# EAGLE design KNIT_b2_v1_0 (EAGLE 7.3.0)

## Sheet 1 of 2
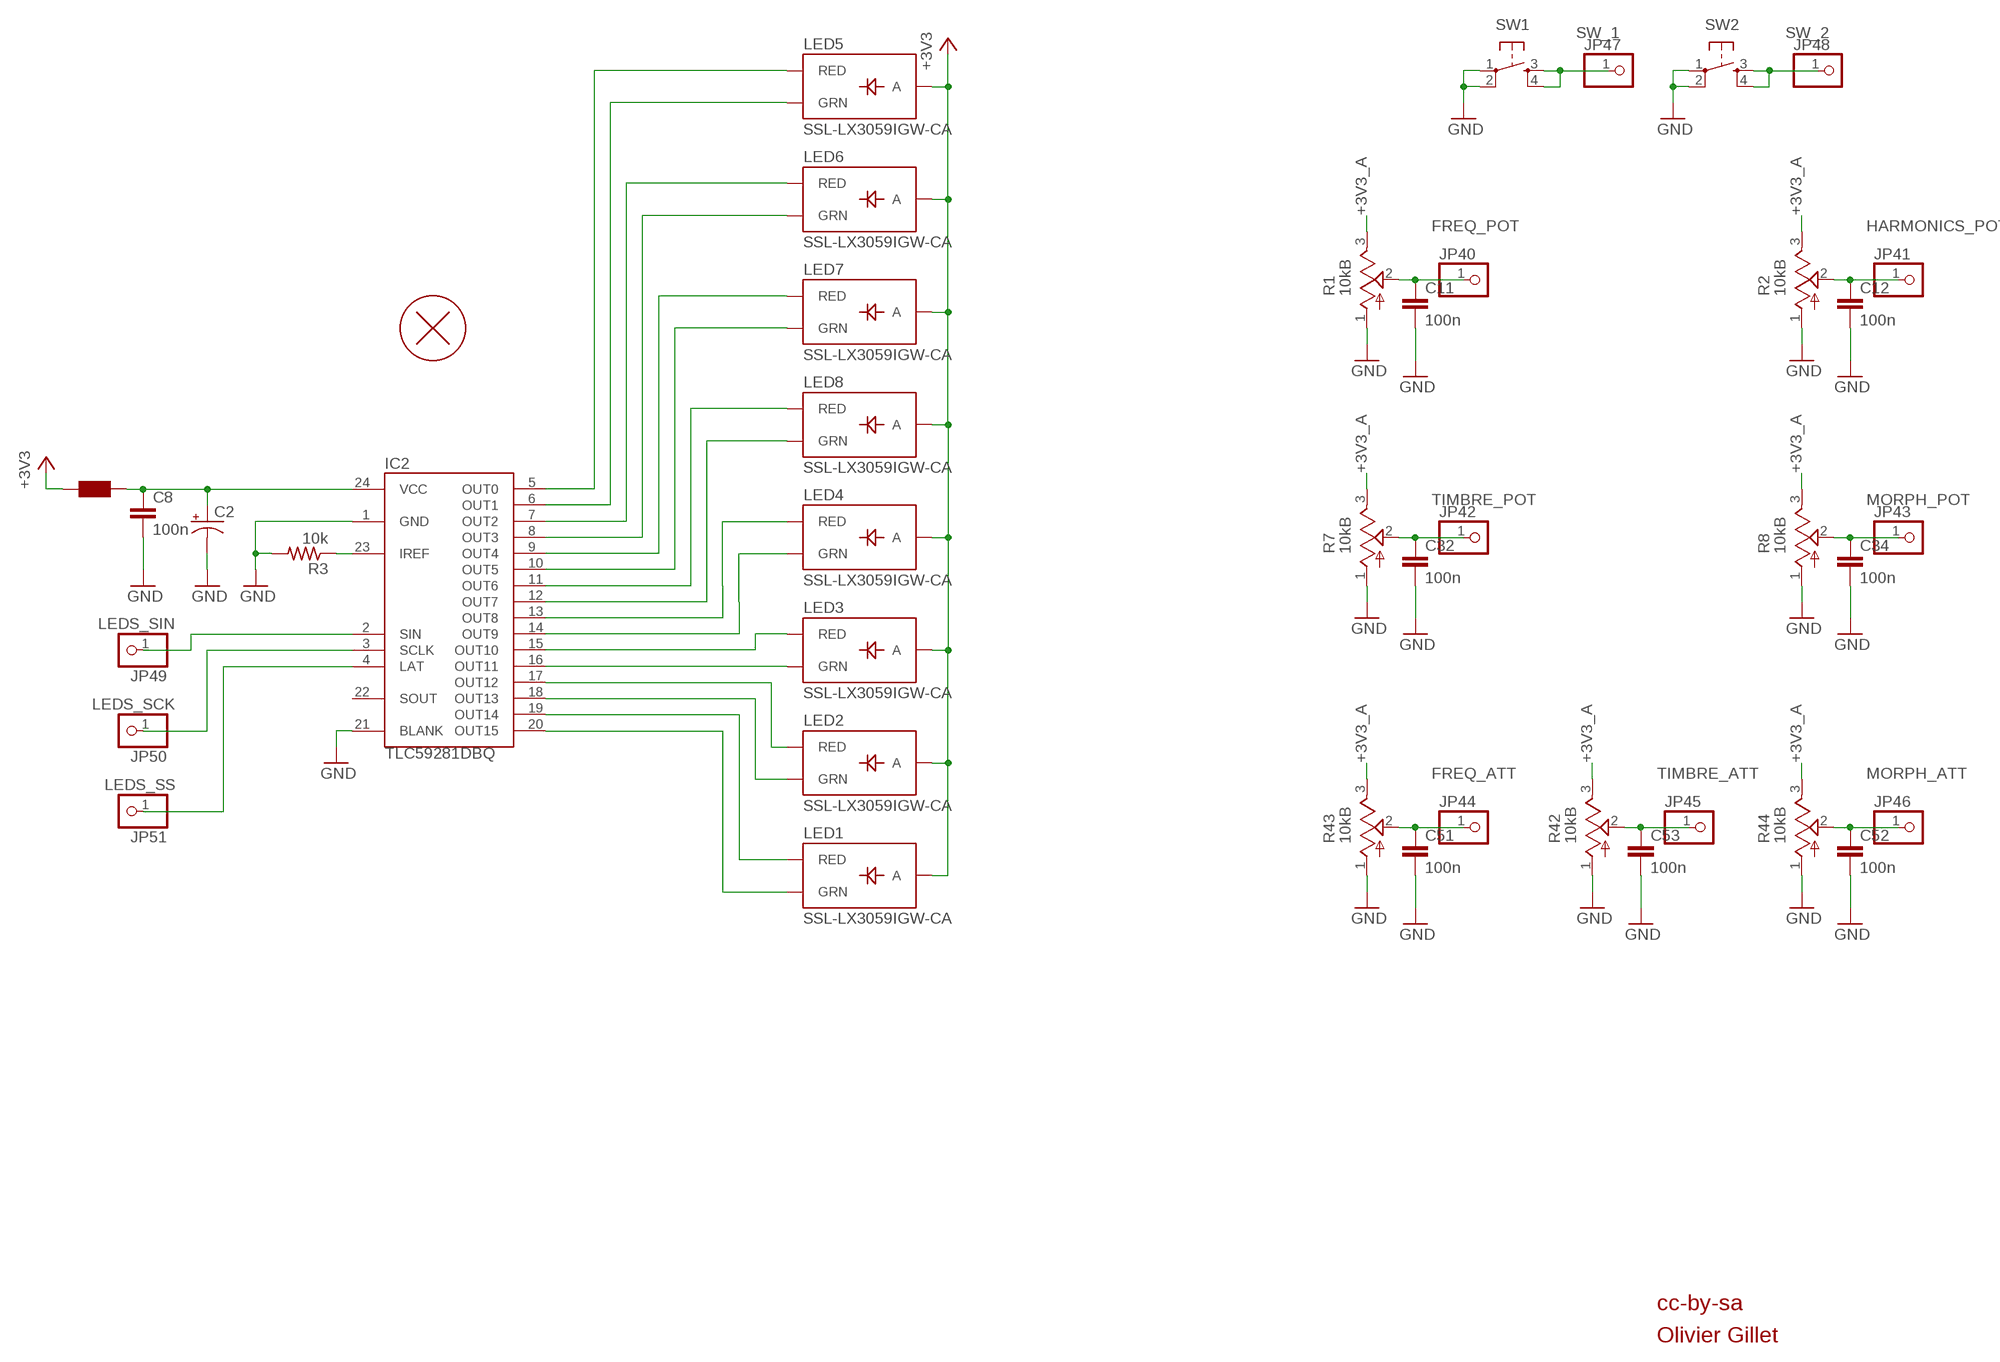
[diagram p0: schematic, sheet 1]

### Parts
C2  CAP_POL  [PANASONIC_B]
C8  100n  CAPACITOR  [RESISTOR_0603]
C11  100n  CAPACITOR  [RESISTOR_0603]
C12  100n  CAPACITOR  [RESISTOR_0603]
C32  100n  CAPACITOR  [RESISTOR_0603]
C34  100n  CAPACITOR  [RESISTOR_0603]
C51  100n  CAPACITOR  [RESISTOR_0603]
C52  100n  CAPACITOR  [RESISTOR_0603]
C53  100n  CAPACITOR  [RESISTOR_0603]
F1  FERRITE-BEAD  [RESISTOR_0603]
H1  PCB_SCREW  [PCB_SCREW]
IC2  TLC59281DBQ  [TSSOP24_0635]
JP40  PINHD-1X1  [1X01]
JP41  PINHD-1X1  [1X01]
JP42  PINHD-1X1  [1X01]
JP43  PINHD-1X1  [1X01]
JP44  PINHD-1X1  [1X01]
JP45  PINHD-1X1  [1X01]
JP46  PINHD-1X1  [1X01]
JP47  PINHD-1X1  [1X01]
JP48  PINHD-1X1  [1X01]
JP49  PINHD-1X1  [1X01]
JP50  PINHD-1X1  [1X01]
JP51  PINHD-1X1  [1X01]
LED1  SSL-LX3059IGW-CA  LED-BICOLOR-THROUGHHOLE-CA  [LED-BICOLOR-THROUGHHOLE-LUMEX]
LED2  SSL-LX3059IGW-CA  LED-BICOLOR-THROUGHHOLE-CA  [LED-BICOLOR-THROUGHHOLE-LUMEX]
LED3  SSL-LX3059IGW-CA  LED-BICOLOR-THROUGHHOLE-CA  [LED-BICOLOR-THROUGHHOLE-LUMEX]
LED4  SSL-LX3059IGW-CA  LED-BICOLOR-THROUGHHOLE-CA  [LED-BICOLOR-THROUGHHOLE-LUMEX]
LED5  SSL-LX3059IGW-CA  LED-BICOLOR-THROUGHHOLE-CA  [LED-BICOLOR-THROUGHHOLE-LUMEX]
LED6  SSL-LX3059IGW-CA  LED-BICOLOR-THROUGHHOLE-CA  [LED-BICOLOR-THROUGHHOLE-LUMEX]
LED7  SSL-LX3059IGW-CA  LED-BICOLOR-THROUGHHOLE-CA  [LED-BICOLOR-THROUGHHOLE-LUMEX]
LED8  SSL-LX3059IGW-CA  LED-BICOLOR-THROUGHHOLE-CA  [LED-BICOLOR-THROUGHHOLE-LUMEX]
R1  10kB  POT_VERTICAL  [ALPS_POT_VERTICAL]
R2  10kB  POT_VERTICAL  [ALPS_POT_VERTICAL]
R3  10k  RESISTOR  [RESISTOR_0603]
R7  10kB  POT_VERTICAL  [ALPS_POT_VERTICAL]
R8  10kB  POT_VERTICAL  [ALPS_POT_VERTICAL]
R42  10kB  POT_VERTICAL  [ALPS_POT_VERTICAL]
R43  10kB  POT_VERTICAL  [ALPS_POT_VERTICAL]
R44  10kB  POT_VERTICAL  [ALPS_POT_VERTICAL]
SW1  TAC_SWITCHPTH  [TACTILE-PTH]
SW2  TAC_SWITCHPTH  [TACTILE-PTH]

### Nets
+3V3: F1.2 LED1.A LED2.A LED3.A LED4.A LED5.A LED6.A LED7.A LED8.A ; also sheet 2
+3V3_A: R1.3(B) R2.3(B) R7.3(B) R8.3(B) R42.3(B) R43.3(B) R44.3(B) ; also sheet 2
FREQ_ATT: C51.1 JP44.1 R43.2(W)
FREQ_POT: C11.1 JP40.1 R1.2(W)
GND: C2.- C8.2 C11.2 C12.2 C32.2 C34.2 C51.2 C52.2 C53.2 IC2.1(GND) IC2.21(BLANK) R1.1(A) R2.1(A) R3.2 R7.1(A) R8.1(A) R42.1(A) R43.1(A) R44.1(A) SW1.1 SW1.2 SW2.1 SW2.2 ; also sheet 2
HARMONICS_POT: C12.1 JP41.1 R2.2(W)
LEDS_SCK: IC2.3(SCLK) JP50.1
LEDS_SIN: IC2.2(SIN) JP49.1
LEDS_SS: IC2.4(LAT) JP51.1
MORPH_ATT: C52.1 JP46.1 R44.2(W)
MORPH_POT: C34.1 JP43.1 R8.2(W)
N$2: IC2.12(OUT7) LED8.GREEN_C(GRN)
N$5: IC2.11(OUT6) LED8.RED_C(RED)
N$9: IC2.10(OUT5) LED7.GREEN_C(GRN)
N$10: IC2.9(OUT4) LED7.RED_C(RED)
N$11: IC2.8(OUT3) LED6.GREEN_C(GRN)
N$12: IC2.13(OUT8) LED4.RED_C(RED)
N$13: IC2.7(OUT2) LED6.RED_C(RED)
N$14: IC2.14(OUT9) LED4.GREEN_C(GRN)
N$15: IC2.6(OUT1) LED5.GREEN_C(GRN)
N$17: IC2.15(OUT10) LED3.RED_C(RED)
N$18: IC2.16(OUT11) LED3.GREEN_C(GRN)
N$19: IC2.17(OUT12) LED2.RED_C(RED)
N$20: IC2.18(OUT13) LED2.GREEN_C(GRN)
N$21: IC2.19(OUT14) LED1.RED_C(RED)
N$22: IC2.5(OUT0) LED5.RED_C(RED)
N$23: IC2.20(OUT15) LED1.GREEN_C(GRN)
N$27: C2.+ C8.1 F1.1 IC2.24(VCC)
N$68: IC2.23(IREF) R3.1
SW_1: JP47.1 SW1.3 SW1.4
SW_2: JP48.1 SW2.3 SW2.4
TIMBRE_ATT: C53.1 JP45.1 R42.2(W)
TIMBRE_POT: C32.1 JP42.1 R7.2(W)
Unconnected: IC2.22(SOUT)

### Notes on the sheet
- cc-by-sa
- Olivier Gillet

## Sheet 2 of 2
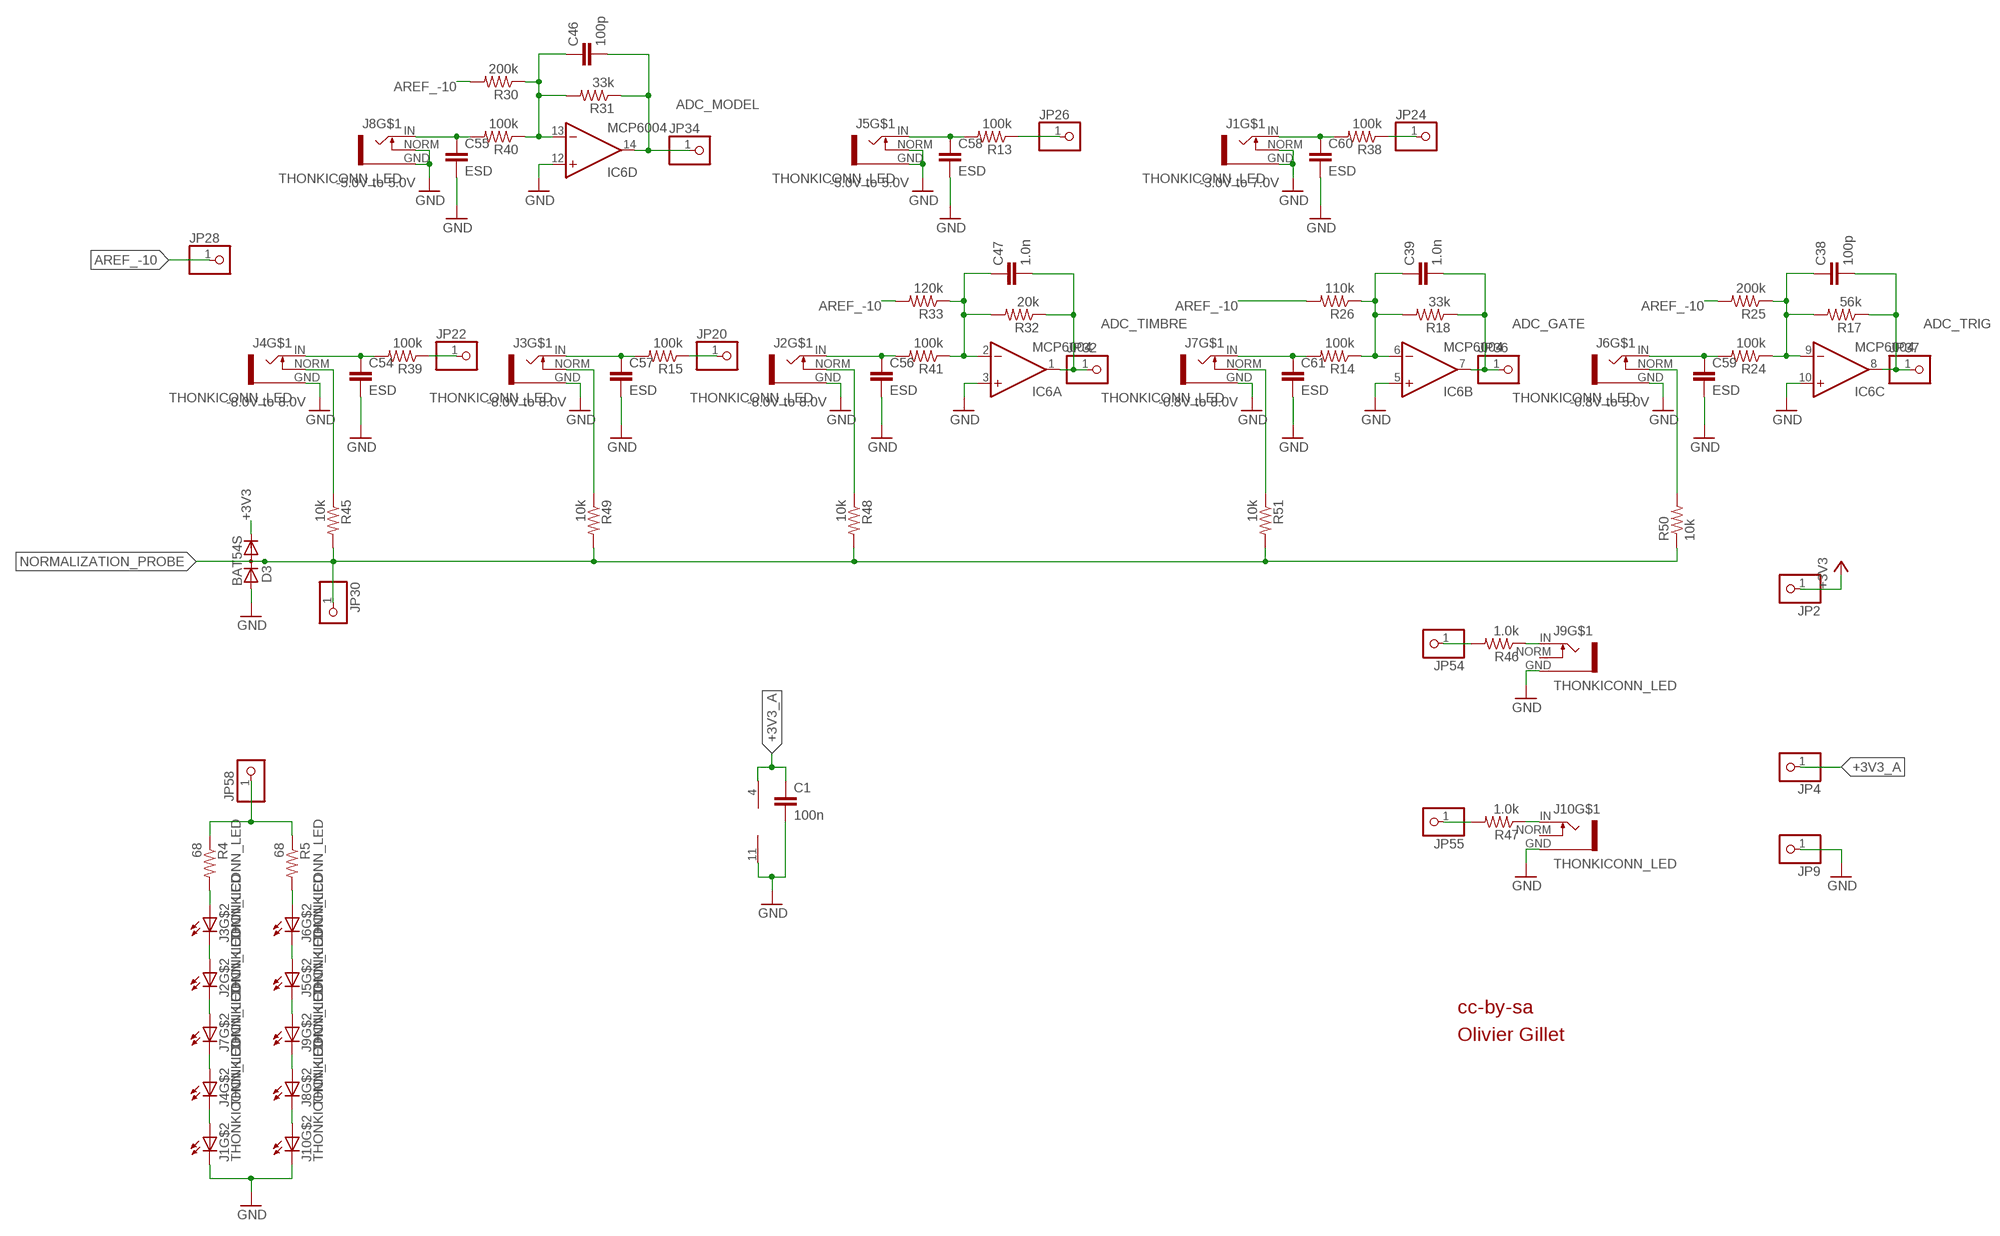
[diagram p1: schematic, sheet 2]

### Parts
C1  100n  CAPACITOR  [RESISTOR_0603]
C38  100p  CAPACITOR  [RESISTOR_0603]
C39  1.0n  CAPACITOR  [RESISTOR_0603]
C46  100p  CAPACITOR  [RESISTOR_0603]
C47  1.0n  CAPACITOR  [RESISTOR_0603]
C54  ESD  CAPACITOR  [RESISTOR_0603]
C55  ESD  CAPACITOR  [RESISTOR_0603]
C56  ESD  CAPACITOR  [RESISTOR_0603]
C57  ESD  CAPACITOR  [RESISTOR_0603]
C58  ESD  CAPACITOR  [RESISTOR_0603]
C59  ESD  CAPACITOR  [RESISTOR_0603]
C60  ESD  CAPACITOR  [RESISTOR_0603]
C61  ESD  CAPACITOR  [RESISTOR_0603]
D3  BAT54S  DIODE_2CACA-SOT23  [SOT23]
IC6  MCP6004  TL074PW  [TSSOP14_065]
J1  THONKICONN_LED  [LED_JACK]
J2  THONKICONN_LED  [LED_JACK]
J3  THONKICONN_LED  [LED_JACK]
J4  THONKICONN_LED  [LED_JACK]
J5  THONKICONN_LED  [LED_JACK]
J6  THONKICONN_LED  [LED_JACK]
J7  THONKICONN_LED  [LED_JACK]
J8  THONKICONN_LED  [LED_JACK]
J9  THONKICONN_LED  [LED_JACK]
J10  THONKICONN_LED  [LED_JACK]
JP2  PINHD-1X1  [1X01]
JP4  PINHD-1X1  [1X01]
JP9  PINHD-1X1  [1X01]
JP20  PINHD-1X1  [1X01]
JP22  PINHD-1X1  [1X01]
JP24  PINHD-1X1  [1X01]
JP26  PINHD-1X1  [1X01]
JP28  PINHD-1X1  [1X01]
JP30  PINHD-1X1  [1X01]
JP32  PINHD-1X1  [1X01]
JP34  PINHD-1X1  [1X01]
JP36  PINHD-1X1  [1X01]
JP37  PINHD-1X1  [1X01]
JP54  PINHD-1X1  [1X01]
JP55  PINHD-1X1  [1X01]
JP58  PINHD-1X1  [1X01]
R4  68  RESISTOR  [RESISTOR_0603]
R5  68  RESISTOR  [RESISTOR_0603]
R13  100k  RESISTOR  [RESISTOR_0603]
R14  100k  RESISTOR  [RESISTOR_0603]
R15  100k  RESISTOR  [RESISTOR_0603]
R17  56k  RESISTOR  [RESISTOR_0603]
R18  33k  RESISTOR  [RESISTOR_0603]
R24  100k  RESISTOR  [RESISTOR_0603]
R25  200k  RESISTOR  [RESISTOR_0603]
R26  110k  RESISTOR  [RESISTOR_0603]
R30  200k  RESISTOR  [RESISTOR_0603]
R31  33k  RESISTOR  [RESISTOR_0603]
R32  20k  RESISTOR  [RESISTOR_0603]
R33  120k  RESISTOR  [RESISTOR_0603]
R38  100k  RESISTOR  [RESISTOR_0603]
R39  100k  RESISTOR  [RESISTOR_0603]
R40  100k  RESISTOR  [RESISTOR_0603]
R41  100k  RESISTOR  [RESISTOR_0603]
R45  10k  RESISTOR  [RESISTOR_0603]
R46  1.0k  RESISTOR  [RESISTOR_0603]
R47  1.0k  RESISTOR  [RESISTOR_0603]
R48  10k  RESISTOR  [RESISTOR_0603]
R49  10k  RESISTOR  [RESISTOR_0603]
R50  10k  RESISTOR  [RESISTOR_0603]
R51  10k  RESISTOR  [RESISTOR_0603]

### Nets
+3V3: D3.2(C) JP2.1 ; also sheet 1
+3V3_A: C1.1 IC6.4(P:V+) JP4.1 ; also sheet 1
ADC_GATE: C39.2 IC6.7(B:OUT) JP36.1 R18.1
ADC_MODEL: C46.2 IC6.14(D:OUT) JP34.1 R31.1
ADC_TIMBRE: C47.2 IC6.1(A:OUT) JP32.1 R32.1
ADC_TRIG: C38.2 IC6.8(C:OUT) JP37.1 R17.1
AREF_-10: JP28.1 R25.2 R26.2 R30.2 R33.2
FM_IN: C57.1 J3.IN R15.2
GATE_IN: C61.1 J7.IN R14.2
GATE_IN1: C59.1 J6.IN R24.2
GND: C1.2 C54.2 C55.2 C56.2 C57.2 C58.2 C59.2 C60.2 C61.2 D3.1(A) IC6.3(A:+IN) IC6.5(B:+IN) IC6.10(C:+IN) IC6.11(P:V-) IC6.12(D:+IN) J1.C J1.GND J1.NORM J2.GND J3.GND J4.GND J5.GND J5.NORM J6.GND J7.GND J8.GND J8.NORM J9.GND J10.C J10.GND JP9.1 ; also sheet 1
HARMONICS_IN: C58.1 J5.IN R13.2
MODEL_IN: C55.1 J8.IN R40.2
MORPH_IN: C54.1 J4.IN R39.2
N$1: J2.A J3.C
N$3: J6.NORM R50.2
N$4: C38.1 IC6.9(C:-IN) R17.2 R24.1 R25.1
N$6: J2.C J7.A
N$7: J4.A J7.C
N$8: J1.A J4.C
N$16: J5.A J6.C
N$24: J3.NORM R49.1
N$25: J2.NORM R48.1
N$26: J4.NORM R45.1
N$28: C39.1 IC6.6(B:-IN) R14.1 R18.2 R26.1
N$29: J5.C J9.A
N$30: J8.A J9.C
N$31: C56.1 J2.IN R41.2
N$32: J8.C J10.A
N$33: J3.A R4.2
N$34: J6.A R5.2
N$35: JP58.1 R4.1 R5.1
N$36: J7.NORM R51.1
N$37: C46.1 IC6.13(D:-IN) R30.1 R31.2 R40.1
N$39: C47.1 IC6.2(A:-IN) R32.2 R33.1 R41.1
N$44: JP20.1 R15.1
N$45: JP22.1 R39.1
N$49: JP24.1 R38.1
N$50: JP26.1 R13.1
N$52: JP54.1 R46.2
N$53: JP55.1 R47.2
N$65: J9.IN R46.1
N$69: J10.IN R47.1
NORMALIZATION_PROBE: D3.3(AC) JP30.1 R45.2 R48.2 R49.2 R50.1 R51.2
V_OCT_IN: C60.1 J1.IN R38.2
Unconnected: J9.NORM J10.NORM

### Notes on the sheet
- -5.0V to 5.0V | -5.0V to 5.0V | -3.0V to 7.0V
- -8.0V to 8.0V | -8.0V to 8.0V | -8.0V to 8.0V | -0.8V to 8.0V | -0.8V to 5.0V
- cc-by-sa
- Olivier Gillet

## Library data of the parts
C1 C8 C11 C12 C32 C34 C38 C39 C46 C47 C51-C61 = parts_aman:CAPACITOR
C2 = parts_aman:CAP_POL
D3 = diode:DIODE_2CACA-: 2 Diodes - Cathode-Anode|Cathode-Anode
F1 = parts_aman:FERRITE-BEAD
H1 = parts_aman:PCB_SCREW
IC2 = og-ics:TLC59281
IC6 = og-linear:TL074: OP AMP
J1-J10 = parts_aman:THONKICONN_LED
JP2 JP4 JP9 JP20 JP22 JP24 JP26 JP28 JP30 JP32 JP34 JP36 JP37 JP40-JP51 JP54 JP55 JP58 = parts_aman:PINHD-1X1: PIN HEADER
LED1-LED8 = og-leds:LED-BICOLOR-THROUGHHOLE-CA
R1 R2 R7 R8 R42-R44 = parts_aman:POT_VERTICAL
R3-R5 R13-R15 R17 R18 R24-R26 R30-R33 R38-R41 R45-R51 = parts_aman:RESISTOR
SW1 SW2 = SparkFun:TAC_SWITCH: Momentary Switch Button commonly used for reset or general input. Spark Fun Electronics SKU : COM-00097

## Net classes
0 default: width 0.152 mm, drill 0.305 mm, clearance 0.152 mm

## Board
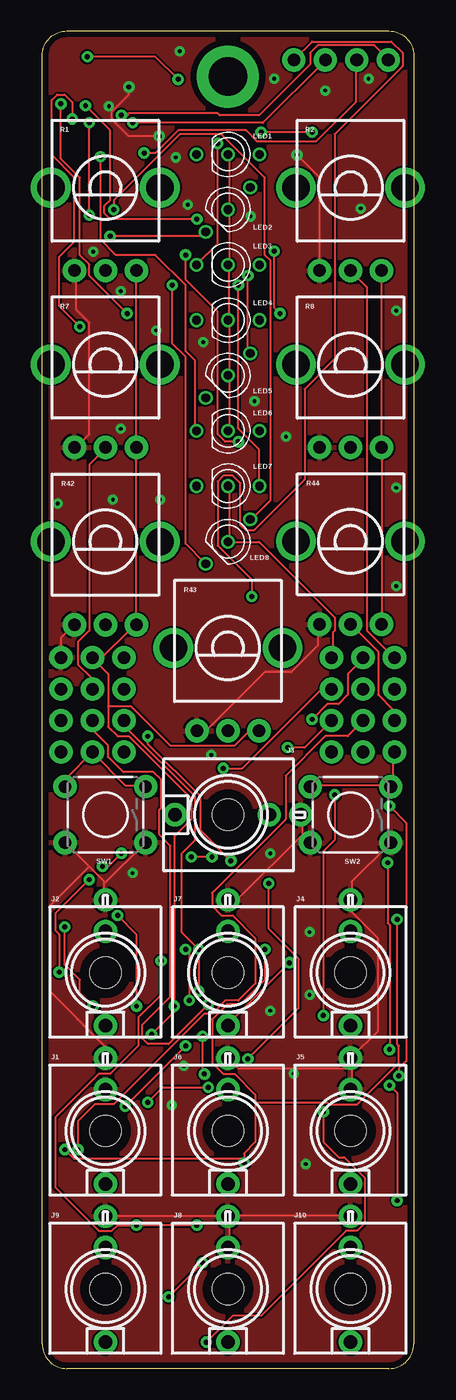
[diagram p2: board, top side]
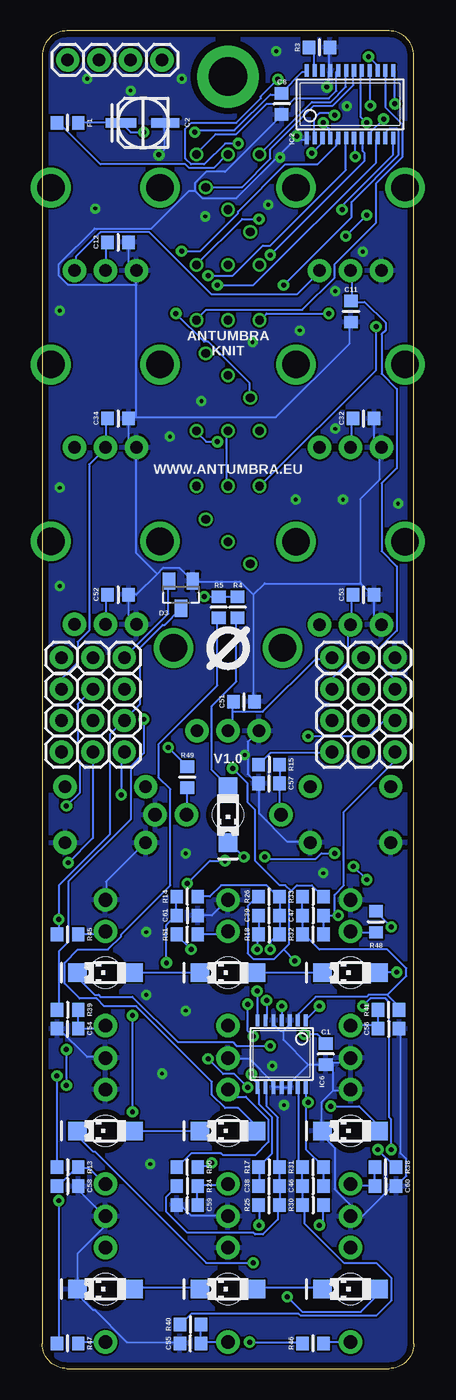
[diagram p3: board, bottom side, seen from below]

Size 30 x 108 mm. Coordinates in mm from the lower left corner, seen from the top.
Outline: 28,0 2,0 arc-90 0,2 0,106 arc-90 2,108 28,108 arc-90 30,106 30,2 arc-90 28,0
Copper layers (1*16): Top 0.035mm / dielectric 1.5mm / Bottom 0.035mm
Design rules "PCBCart-Standard *": minimum track width 6mil, minimum drill 0.4mm, track to track 6mil, track to pad 6mil, pad to pad 6mil, via to via 6mil, smd to smd 6mil, copper to edge 20mil, drill to drill 8mil, minimum pad ring 8mil, minimum via ring 10mil, stop-mask expansion 3mil, vias tented up to drill 25mil, thermal gap 8mil

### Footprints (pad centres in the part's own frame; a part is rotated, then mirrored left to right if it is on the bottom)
RESISTOR_0603 = smd 1 x 1.1: 1 -0.85,0; 2 0.85,0
PANASONIC_B = smd 2.464 x 0.762: + 1.778,0 | smd 2.286 x 0.762: - -1.778,0
SOT23 = smd 1 x 1.4: 1 -0.95,-1.1; 2 0.95,-1.1; 3 0,1.1
PCB_SCREW = drill 3.1 pad 5: P$1 0,0
TSSOP24_0635 = smd 0.33 x 1: 1 -3.493,-2.725; 2 -2.857,-2.725; 3 -2.223,-2.725; 4 -1.587,-2.725; 5 -0.953,-2.725; 6 -0.318,-2.725; 7 0.318,-2.725; 8 0.953,-2.725; 9 1.587,-2.725; 10 2.223,-2.725; 11 2.857,-2.725; 12 3.493,-2.725; 13 3.493,2.725; 14 2.857,2.725; 15 2.223,2.725; 16 1.587,2.725; 17 0.953,2.725; 18 0.318,2.725; 19 -0.318,2.725; 20 -0.953,2.725; 21 -1.587,2.725; 22 -2.223,2.725; 23 -2.857,2.725; 24 -3.493,2.725
TSSOP14_065 = smd 0.305 x 0.991: 1 -1.95,-2.718; 2 -1.3,-2.718; 3 -0.65,-2.718; 4 0,-2.718; 5 0.65,-2.718; 6 1.3,-2.718; 7 1.95,-2.718; 8 1.95,2.718; 9 1.3,2.718; 10 0.65,2.718; 11 0,2.718; 12 -0.65,2.718; 13 -1.3,2.718; 14 -1.95,2.718
LED_JACK = smd 1.5 x 1.5 bottom: A 2.266,0; C -2.266,0 | drill 1.1 pad 1.88: GND 0,-5.88; IN 0,4.28; NORM 0,-3.34 | hole 2.5: 0,0
1X01 = drill 1.016 pad 1.88: 1 0,0
LED-BICOLOR-THROUGHHOLE-LUMEX = drill 0.7: A 0,0; GREEN_C 2.54,0; RED_C -2.54,0
ALPS_POT_VERTICAL = drill 1 pad 1.88: 1 -2.5,-6.7; 2 0,-6.7; 3 2.5,-6.7 | drill 2.2 pad 3.175: P$4 4.4,0; P$5 -4.4,0
TACTILE-PTH = drill 1.016 pad 1.88: 1 -3.251,2.261; 2 3.251,2.261; 3 -3.251,-2.261; 4 3.251,-2.261

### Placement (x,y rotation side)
C1  7.11,25.4 270 bottom
C2  21.84,100.58 180 bottom
C8  10.67,102.11 270 bottom
C11  5.08,85.34 270 bottom
C12  23.88,90.93 0 bottom
C32  4.06,76.71 0 bottom
C34  23.88,76.71 0 bottom
C38  11.68,14.73 180 bottom
C39  11.68,36.58 180 bottom
C46  8.13,14.73 0 bottom
C47  8.13,36.58 0 bottom
C51  13.72,53.85 0 bottom
C52  23.88,62.48 0 bottom
C53  4.06,62.48 0 bottom
C54  27.94,27.43 180 bottom
C55  18.03,2.03 180 bottom
C56  2.03,27.43 0 bottom
C57  11.68,47.24 180 bottom
C58  27.94,14.73 0 bottom
C59  18.29,13.21 180 bottom
C60  2.29,14.73 0 bottom
C61  18.29,36.58 0 bottom
D3  18.8,62.48 180 bottom
F1  27.94,100.58 180 bottom
H1  15,104.31 0 top
IC2  5.15,102.08 0 bottom
IC6  10.67,25.4 180 bottom
J1  5.11,19.19 180 top
J2  5.11,31.96 180 top
J3  15,44.71 90 top
J4  24.89,31.96 180 top
J5  24.89,19.19 180 top
J6  15,19.19 180 top
J7  15,31.96 180 top
J8  15,6.42 180 top
J9  5.11,6.42 180 top
J10  24.89,6.42 180 top
JP2  23.37,57.4 0 bottom
JP4  4.06,57.4 0 bottom
JP9  1.52,57.4 0 bottom
JP20  6.6,49.78 0 bottom
JP22  25.91,57.4 0 bottom
JP24  25.91,52.32 0 bottom
JP26  25.91,54.86 0 bottom
JP28  23.37,54.86 0 bottom
JP30  23.37,52.32 0 bottom
JP32  1.52,49.78 0 bottom
JP34  1.52,52.32 0 bottom
JP36  6.6,52.32 0 bottom
JP37  4.06,52.32 0 bottom
JP40  1.52,54.86 0 bottom
JP41  28.45,57.4 0 bottom
JP42  4.06,54.86 0 bottom
JP43  28.45,54.86 0 bottom
JP44  6.6,57.4 0 bottom
JP45  6.6,54.86 0 bottom
JP46  28.45,52.32 0 bottom
JP47  4.06,49.78 0 bottom
JP48  28.45,49.78 0 bottom
JP49  27.94,105.66 0 bottom
JP50  25.4,105.66 0 bottom
JP51  22.86,105.66 0 bottom
JP54  23.37,49.78 0 bottom
JP55  25.91,49.78 0 bottom
JP58  20.32,105.66 0 bottom
LED1  15,98.04 0 top
LED2  15,93.58 45 top
LED3  15,89.11 0 top
LED4  15,84.65 0 top
LED5  15,80.18 45 top
LED6  15,75.72 0 top
LED7  15,71.26 0 top
LED8  15,66.76 45 top
R1  5.11,95.35 0 top
R2  24.89,95.35 0 top
R3  7.62,106.68 0 bottom
R4  14.22,61.47 270 bottom
R5  15.75,61.47 270 bottom
R7  5.11,81.07 0 top
R8  24.89,81.07 0 top
R13  27.94,16.26 0 bottom
R14  18.29,38.1 180 bottom
R15  11.68,48.77 0 bottom
R17  11.68,16.26 0 bottom
R18  11.68,35.05 0 bottom
R24  18.29,14.73 0 bottom
R25  11.68,13.21 180 bottom
R26  11.68,38.1 180 bottom
R30  8.13,13.21 0 bottom
R31  8.13,16.26 180 bottom
R32  8.13,35.05 180 bottom
R33  8.13,38.1 0 bottom
R38  2.29,16.26 180 bottom
R39  27.94,28.96 0 bottom
R40  18.03,3.56 0 bottom
R41  2.03,28.96 180 bottom
R42  5.11,66.76 0 top
R43  15,58.19 0 top
R44  24.89,66.79 0 top
R45  27.94,35.05 180 bottom
R46  8.13,2.03 180 bottom
R47  27.94,2.03 180 bottom
R48  3.05,36.07 90 bottom
R49  18.29,47.75 90 bottom
R50  18.29,16.26 180 bottom
R51  18.29,35.05 180 bottom
SW1  5.11,44.73 180 top
SW2  24.89,44.71 180 top
U$1  [LOGO_3.5]  14.99,58.17 0 bottom

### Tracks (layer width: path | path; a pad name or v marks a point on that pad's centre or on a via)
+3V3
  Top 0.152: LED7.A 15.09,71.17 15.09,66.9 LED8.A 15.09,66.75 17.53,66.75 23.62,60.66 23.62,59.59 23.47,59.44 23.47,57.45 JP2.1 | LED1.A 15.09,97.99 15.09,93.73 LED2.A 15.09,93.57 15.09,89.15 LED3.A 15.09,89 15.09,84.73 LED4.A 15.09,84.58 15.09,80.31 LED5.A 15.09,80.16 15.09,75.74 LED6.A
  Bottom 0.152: JP2.1 19.81,60.96 19.81,63.55 D3.2 | LED6.A 15.09,75.59 15.09,71.32 LED7.A | F1.2 28.65,100.58 25.3,97.23 18.44,97.23 18.14,96.93 16.15,96.93 15.09,97.99 LED1.A
+3V3_A  (via drill 0.4)
  Top 0.152: R44.3 27.43,60.2 27.43,74.22 R8.3 27.43,74.37 27.43,88.54 R2.3 | v8.84,26.98 10.67,28.8 v10.67,29.26 10.67,42.98 12.04,44.35 12.04,46.02 7.01,51.05 6.1,51.05 5.33,51.82 5.33,53.49 | 5.33,53.49 5.33,56.08 4.42,57 | 4.42,57 4.12,57.3 JP4.1 4.42,57 | 4.42,57 7.47,60.05 R42.3 7.62,60.2 7.62,74.22 R7.3 7.62,88.54 R1.3 | 5.33,53.49 7.16,53.49 10.36,50.29 15.54,50.29 16.61,51.36 17.37,51.36 R43.3
  Bottom 0.152: v10.67,29.26 IC6.4 | v8.84,26.98 7.77,26.98 7.16,26.36 C1.1 | R2.3 27.28,88.7 27.28,89.76 25.3,91.75 21.34,91.75 16.31,86.72 9.45,86.72 7.62,88.54 R1.3
ADC_GATE  (via drill 0.4)
  Top 0.152: v12.65,30.48 v12.65,33.83 11.28,35.2 11.28,41.6 12.34,42.67 12.34,46.18 6.71,51.82 6.71,52.27 JP36.1
  Bottom 0.152: v12.65,30.48 12.65,28.19 IC6.7 | v12.65,33.83 12.65,35.05 R18.1 12.5,35.05 12.5,36.58 C39.2
ADC_MODEL  (via drill 0.4)
  Top 0.152: v8.53,51.05 8.53,50.44 12.8,46.18 12.8,43.43 v15.24,41 | v18.29,39.17 18.29,35.51 20.73,33.07 20.73,29.11 v16.61,24.99 | v13.41,22.71 9.75,22.71 v8.53,21.49
  Bottom 0.152: 8.69,21.49 8.69,17.68 7.32,16.31 R31.1 7.32,16.15 7.32,14.78 C46.2 | 8.69,21.49 8.69,22.55 IC6.14 | v8.53,51.05 3.66,51.05 2.44,52.27 1.52,52.27 JP34.1 | v15.24,41 16.46,41 v18.29,39.17 | v16.61,24.99 15.39,23.77 14.48,23.77 v13.41,22.71 | 8.69,21.49 v8.53,21.49
ADC_TIMBRE  (via drill 0.4)
  Top 0.152: v7.62,29.26 7.62,35.05 v6.1,36.58
  Bottom 0.152: v7.62,29.26 8.69,28.19 IC6.1 | 6.4,36.58 C47.2 7.32,36.58 7.32,35.05 R32.1 | JP32.1 1.52,49.07 5.64,44.96 5.64,39.01 6.4,38.25 6.4,36.58 | 6.4,36.58 v6.1,36.58
ADC_TRIG  (via drill 0.4)
  Top 0.152: v13.41,29.41 10.21,26.21 8.53,26.21 8.08,26.67 8.08,27.74 10.36,30.02 10.36,42.22 9.45,43.13 9.45,45.11 9.6,45.26 9.6,47.55 8.99,48.16 6.55,48.16 5.33,49.38 5.33,50.29 4.12,51.51 4.12,52.27 JP37.1 | v12.95,26.82 12.95,23.93 v13.11,23.77
  Bottom 0.152: C38.2 12.5,14.78 12.5,16.15 R17.1 12.5,16.31 11.43,17.37 11.43,20.27 12.5,21.34 12.5,22.55 IC6.8 12.65,22.71 12.65,23.01 13.11,23.47 v13.11,23.77 | v13.41,29.41 13.41,27.28 v12.95,26.82
AREF_-10  (via drill 0.4)
  Top 0.152: v12.5,11.58 v7.62,11.58 6.1,11.58 5.64,11.12 4.57,11.12 1.07,14.63 1.07,20.27 4.57,23.77 5.49,23.77 7.77,26.06 7.77,28.35 9.6,30.18 v9.6,32.92 | JP28.1 22.55,54.86 16.15,48.46 v14.63,48.46
  Bottom 0.152: v7.62,11.58 7.32,11.89 7.32,13.11 R30.2 | v12.5,11.58 12.5,13.11 R25.2 | 9.91,38.56 10.06,38.41 10.06,34.29 10.52,33.83 | 9.91,38.56 9.45,39.01 8.23,39.01 7.32,38.1 R33.2 | 10.52,33.83 11.28,33.07 12.95,33.07 13.41,33.53 13.41,37.34 12.65,38.1 R26.2 | 10.52,33.83 v9.6,32.92 | v14.63,48.46 13.41,47.24 13.41,45.72 12.8,45.11 12.8,41 10.82,39.01 10.36,39.01 9.91,38.56
FM_IN
  Bottom 0.152: C57.1 R15.2 | C57.1 10.82,44.81 J3.IN | C57.1
FREQ_ATT
  Bottom 0.152: 14.63,53.03 14.63,51.82 14.94,51.51 R43.2 | 14.63,53.03 14.63,53.8 C51.1 | 14.63,53.03 12.19,53.03 7.92,57.3 6.71,57.3 JP44.1
FREQ_POT
  Bottom 0.152: R1.2 5.03,88.54 5.03,86.26 C11.1 5.03,86.11 3.96,86.11 2.29,84.43 2.29,83.82 2.59,83.52 2.59,80.31 1.37,79.1 1.37,72.69 2.59,71.48 2.59,65.99 1.37,64.77 1.37,59.59 2.74,58.22 2.74,56.84 1.52,55.63 JP40.1
GATE_IN  (via drill 0.4)
  Top 0.152: v19.96,32.77 14.94,27.74 J7.IN
  Bottom 0.152: 19.2,36.58 19.2,38.1 R14.2 | 19.2,36.58 19.96,35.81 v19.96,32.77 | 19.2,36.58 C61.1
GATE_IN1
  Bottom 0.152: C59.1 17.53,13.26 17.53,14.63 R24.2 17.37,14.78 15.09,14.78 J6.IN
GND  (via drill 0.3, 0.4)
  Top 0.152: SW2.1 28.04,42.37 24.99,39.32 24.99,37.95 J4.GND 24.99,37.8 24.99,36.88 27.13,34.75 27.13,27.28 24.99,25.15 J5.GND | 21.03,43.13 21.03,44.65 J3.GND | 21.03,43.13 21.64,42.52 SW2.2 21.03,43.13 | 21.03,43.13 15.85,37.95 15.09,37.95 J7.GND | J8.NORM 15.09,9.91 15.09,12.19 J8.GND | J8.GND 15.09,12.34 24.84,12.34 J10.GND | 24.99,24.23 24.99,24.99 J5.GND | 24.99,24.23 24.99,22.55 J5.NORM | 24.99,24.23 15.85,24.23 15.09,24.99 J6.GND | 24.99,24.23 J5.GND | J8.GND 14.94,12.34 5.18,12.34 J9.GND | v7.01,103.48 7.01,102.87 5.64,101.5 5.64,100.89 7.01,99.52 v9.45,99.52 | v20.57,97.99 22.4,96.16 22.4,88.7 R2.1 | 3.81,40.54 5.03,39.32 5.03,39.17 | 3.81,40.54 1.98,42.37 SW1.2 | 5.03,39.17 5.03,37.95 J2.GND | 5.03,39.17 8.23,42.37 SW1.1 | R1.1 2.74,88.54 2.74,85.5 3.81,84.43 3.81,75.44 2.74,74.37 R7.1 | JP9.1 1.52,58.98 2.59,60.05 R42.1 | R43.1 12.65,51.51 13.26,51.51 17.98,56.24 20.12,56.24 22.25,58.37 22.25,60.05 R44.1 | 3.81,40.54 0.61,37.34 0.61,30.48 5.03,26.06 5.03,25.15 J1.GND
  Bottom 0.152: C61.2 16.31,36.58 15.09,37.8 J7.GND | J4.GND 24.84,37.95 24.84,39.32 21.79,42.37 SW2.2 | C59.2 19.05,13.11 18.75,13.11 17.98,12.34 15.09,12.34 J8.GND | C58.2 26.98,14.63 26.98,14.33 24.99,12.34 J10.GND 24.99,12.19 24.99,11.43 27.13,9.3 27.13,6.55 J10.C 27.13,6.4 27.13,5.94 25.91,4.72 25.76,4.72 23.16,2.13 18.9,2.13 C55.2 | C56.2 1.07,27.43 1.07,17.37 0.61,16.92 0.61,15.54 1.37,14.78 C60.2 1.52,14.63 1.83,14.63 4.12,12.34 5.03,12.34 J9.GND 5.18,12.34 5.18,13.26 6.4,14.48 6.4,17.83 7.32,18.75 7.32,19.05 J1.C 7.47,19.2 7.47,21.49 6.55,22.4 | C54.2 28.65,27.43 26.36,25.15 24.99,25.15 J5.GND | 6.55,22.4 5.18,22.4 J1.NORM | 10.52,27.28 10.06,27.74 10.06,28.04 IC6.3 | 10.52,27.28 10.82,27.28 11.28,27.74 11.28,28.04 IC6.5 | 10.67,22.71 10.06,22.71 IC6.12 9.91,22.71 9.91,23.16 8.53,24.54 | 10.67,22.71 11.28,22.71 IC6.10 11.43,22.71 11.43,23.16 13.26,24.99 14.94,24.99 J6.GND | 10.67,22.71 IC6.11 | 6.55,24.69 5.49,24.69 5.18,24.99 J1.GND | 6.55,24.69 7.01,24.69 C1.2 7.16,24.54 8.53,24.54 | 10.52,27.28 10.52,26.52 8.53,24.54 | 6.55,24.69 6.55,22.4 | R3.2 6.86,106.68 6.86,104.85 IC2.21 6.86,104.7 6.86,103.63 v7.01,103.48 | 9.45,99.21 9.6,99.21 14.33,94.49 17.07,94.49 17.68,95.1 | 9.45,99.21 8.69,99.21 IC2.1 | 17.68,95.1 17.68,95.71 16.76,96.62 15.24,96.62 10.67,101.19 C8.2 | 9.45,99.21 v9.45,99.52 | C12.2 23.01,90.83 23.01,89.31 22.4,88.7 R2.1 22.4,88.54 22.4,87.48 | v20.57,97.99 20.12,98.45 20.12,100.58 C2.- | 22.4,76.81 23.01,76.81 C34.2 23.01,76.66 23.01,74.98 22.4,74.37 R8.1 22.4,74.22 22.4,65.84 20.73,64.16 | 22.4,76.81 11.12,76.81 5.18,82.75 5.18,84.43 C11.2
  Bottom 0.152: 22.4,76.81 22.4,87.48 | 17.68,95.1 18.14,95.1 21.18,92.05 25.76,92.05 28.65,89.15 28.65,88.24 27.89,87.48 22.4,87.48 | R43.1 12.65,51.36 13.41,50.6 13.41,48.01 12.65,47.24 C57.2 12.5,47.24 12.5,44.81 10.21,42.52 8.38,42.52 SW1.1 | C32.2 3.2,76.66 3.2,74.83 2.74,74.37 R7.1 2.74,74.22 2.74,71.78 4.27,70.26 4.27,63.4 | R42.1 2.74,60.2 3.2,60.66 C53.2 3.35,62.48 4.27,63.4 | 23.01,62.48 23.01,60.81 22.4,60.2 R44.1 | 12.95,62.48 12.95,53.95 C51.2 | 12.95,62.48 14.02,63.55 17.83,63.55 D3.1 17.98,63.7 18.9,64.62 20.27,64.62 20.73,64.16 | 23.01,62.48 22.4,62.48 20.73,64.16 | 23.01,62.48 C52.2 | 4.27,63.4 12.04,63.4 12.95,62.48
  other vias: 21.27,16.51 20.32,23.81 11.43,24.45 10.48,21.27 21.59,35.24 21.59,30.16 18.41,28.89 18.41,41.59 7.3,40.01 13.65,49.53 5.71,70.17 9.53,70.17 19.68,75.25 28.57,71.12 28.57,63.18 17.14,78.11 28.57,85.41 9.21,83.82 16.83,93.03 25.72,93.66 22.86,103.19 11.11,106.36 5.4,101.92 10.79,97.79 11.75,93.98 18.73,104.14 26.35,104.14 13.02,82.87 4.13,90.17 6.35,75.88 1.27,69.85 6.35,87
  pour Top: 0,0 30,0 30,108 0,108
  pour Bottom: 0,0 30,0 30,108 0,108
HARMONICS_IN
  Bottom 0.152: C58.1 28.65,14.78 27.13,16.31 R13.2 26.98,16.15 26.21,16.15 24.99,14.94 J5.IN
HARMONICS_POT
  Top 0.152: JP41.1 28.35,57.45 26.21,59.59 26.21,87.33 24.99,88.54 R2.2
  Bottom 0.152: C12.1 24.84,90.83 24.84,88.7 R2.2
LEDS_SCK  (via drill 0.4)
  Top 0.152: v8.23,98.15 9.14,98.15 10.97,99.97 16.46,99.97 17.37,99.06 22.1,99.06 25.3,102.26 25.3,105.61 JP50.1
  Bottom 0.152: v8.23,98.15 7.47,98.91 7.47,99.21 IC2.3
LEDS_SIN  (via drill 0.4)
  Top 0.152: v6.4,101.19 6.86,101.19 7.01,101.35 14.17,101.35 14.33,101.19 17.53,101.19 21.64,105.31 21.64,106.22 22.25,106.83 26.82,106.83 27.89,105.77 JP49.1
  Bottom 0.152: v6.4,101.19 6.55,101.35 7.62,101.35 8.08,100.89 8.08,99.36 IC2.2
LEDS_SS  (via drill 0.4)
  Top 0.152: v7.32,100.58 17.83,100.58 22.86,105.61 JP51.1
  Bottom 0.152: v7.32,100.58 6.86,100.13 6.86,99.36 IC2.4
MODEL_IN
  Bottom 0.152: R40.2 17.22,3.5 17.22,2.13 C55.1 17.07,2.13 15.09,2.13 J8.IN
MORPH_ATT
  Top 0.152: JP46.1 28.35,52.43 28.35,53.19 27.13,54.41 27.13,57.91 24.99,60.05 R44.2
  Bottom 0.152: C52.1 24.84,62.48 24.84,60.2 R44.2
MORPH_IN
  Bottom 0.152: R39.2 27.13,28.96 27.13,27.43 C54.1 25.15,27.43 24.99,27.58 J4.IN
MORPH_POT
  Bottom 0.152: C34.1 24.84,76.66 24.84,74.37 R8.2 24.99,74.22 26.21,73 26.21,59.59 27.13,58.67 27.13,57 28.35,55.78 28.35,54.86 JP43.1
N$1  (via drill 0.4)
  Top 0.152: v1.37,32 1.37,35.05 1.07,35.36 1.07,36.73 v3.81,39.47 | v4.88,40.54 5.33,40.54 v6.4,41.6 | v13.72,41.3 v12.04,41.3
  Bottom 0.152: v1.37,32 2.74,32 J2.A | v4.88,40.54 v3.81,39.47 | v6.4,41.6 7.47,41.6 7.92,41.15 11.89,41.15 v12.04,41.3 | v13.72,41.3 14.94,42.52 J3.C
N$2  (via drill 0.4)
  Top 0.152: v5.79,93.57 5.79,94.34 11.12,99.67 14.48,99.67 17.98,96.16 17.98,89.92 18.44,89.46 18.44,70.1 16.92,68.58 LED8.GREEN_C
  Bottom 0.152: v5.79,93.57 5.79,93.88 1.68,97.99 1.68,99.21 IC2.12
N$3
  Bottom 0.152: R50.2 19.05,16.31 17.98,17.37 15.54,17.37 15.39,17.22 12.8,17.22 11.73,18.29 11.73,20.12 13.56,21.95 14.48,21.95 14.94,22.4 J6.NORM
N$4
  Bottom 0.152: IC6.9 11.89,22.55 11.89,21.18 10.97,20.27 10.97,16.31 R17.2 10.82,16.15 10.82,14.78 C38.1 10.82,14.63 10.82,13.26 R25.1 10.97,13.11 10.97,12.04 12.19,10.82 12.8,10.82 12.95,10.97 18.29,10.97 19.96,12.65 19.96,13.87 19.2,14.63 R24.1
N$5  (via drill 0.4)
  Top 0.152: v10.52,87.48 10.52,82.75 11.58,81.69 11.58,66.6 13.11,65.08 LED8.RED_C
  Bottom 0.152: v10.52,87.48 5.03,92.96 5.03,94.18 1.22,97.99 1.22,99.97 1.37,100.13 1.98,100.13 2.29,99.82 IC2.11
N$6
  Bottom 0.152: J2.C 7.47,32 12.65,32 J7.A
N$7
  Bottom 0.152: J7.C 17.37,32 22.55,32 J4.A
N$8  (via drill 0.4)
  Top 0.152: v11.58,26.06 v6.71,21.18
  Bottom 0.152: v6.71,21.18 4.42,21.18 2.9,19.66 2.9,19.2 J1.A | v11.58,26.06 14.33,26.06 14.63,26.36 19.05,26.36 22.71,30.02 25.3,30.02 25.45,30.18 25.76,30.18 27.13,31.55 27.13,31.85 J4.C
N$9  (via drill 0.4)
  Top 0.152: v15.85,87.48 15.85,75.89 17.53,74.22 17.53,71.32 LED7.GREEN_C
  Bottom 0.152: v15.85,87.48 12.95,87.48 3.05,97.38 3.05,99.21 IC2.10
N$10  (via drill 0.4)
  Top 0.152: v2.44,100.89 2.44,102.26 1.83,102.87 1.22,102.87 0.76,102.41 0.76,97.99 2.59,96.16 2.59,90.98 1.37,89.76 1.37,85.8 v3.05,84.12
  Bottom 0.152: v2.44,100.89 3.5,99.82 3.5,99.36 IC2.9 | v3.05,84.12 3.05,80.62 12.34,71.32 LED7.RED_C
N$11  (via drill 0.4)
  Top 0.152: v11.58,89.92 11.58,87.94 14.17,85.34 14.17,75.44 14.78,74.83 v15.85,74.83
  Bottom 0.152: v11.58,89.92 3.96,97.54 3.96,98.15 4.12,98.3 4.12,99.21 IC2.8 | v15.85,74.83 16.76,74.83 17.53,75.59 LED6.GREEN_C
N$12  (via drill 0.4)
  Top 0.152: v1.52,102.11 1.52,97.69 3.05,96.16 3.05,89.92 3.81,89.15 3.81,88.24 v6.86,85.19
  Bottom 0.152: v1.52,102.11 1.52,104.7 IC2.13 | v6.86,85.19 11.89,85.19 12.34,84.73 LED4.RED_C
N$13  (via drill 0.4)
  Top 0.152: v4.72,97.84 4.72,91.14 5.94,89.92 9.14,89.92 11.58,87.48 11.58,82.14 12.34,81.38 12.34,75.74 LED6.RED_C
  Bottom 0.152: v4.72,97.84 4.72,99.21 IC2.7
N$14
  Bottom 0.152: IC2.14 2.29,104.7 2.29,101.8 0.91,100.43 0.91,97.84 3.05,95.71 3.05,92.51 6.4,89.15 6.4,88.09 8.99,85.5 16.76,85.5 17.53,84.73 LED4.GREEN_C
N$15  (via drill 0.4)
  Top 0.152: v16.61,88.24 16.61,82.14 16.76,81.99 LED5.GREEN_C
  Bottom 0.152: v16.61,88.24 14.63,88.24 12.19,90.68 11.58,90.68 5.49,96.77 5.49,99.21 IC2.6
N$16
  Bottom 0.152: J6.C 17.37,19.2 22.55,19.2 J5.A
N$17  (via drill 0.4)
  Top 0.152: v3.66,105.92 9.14,105.92 v10.97,104.09 | v14.17,98.91 14.17,90.83 12.5,89.15 LED3.RED_C
  Bottom 0.152: v3.66,105.92 3.05,105.31 3.05,104.85 IC2.15 | v10.97,104.09 12.34,102.72 12.34,102.56 14.33,100.58 17.98,100.58 18.44,100.13 18.44,97.69 17.98,97.23 16.92,97.23 15.24,98.91 v14.17,98.91
N$18  (via drill 0.4)
  Top 0.152: v3.5,101.96 5.49,99.97 5.49,94.34 5.03,93.88 5.03,93.27 5.49,92.81 v12.5,92.81
  Bottom 0.152: v3.5,101.96 3.5,104.7 IC2.16 | v12.5,92.81 13.87,92.81 17.53,89.15 LED3.GREEN_C
N$19  (via drill 0.4)
  Top 0.152: v3.81,93.12 v3.81,100.58 | v5.49,91.44 12.8,91.44 13.11,91.75 LED2.RED_C
  Bottom 0.152: v3.81,100.58 4.27,101.04 4.27,104.7 IC2.17 | v5.49,91.44 v3.81,93.12
N$20
  Bottom 0.152: IC2.18 4.88,104.7 4.88,103.63 6.55,101.96 8.08,101.96 11.58,98.45 11.58,97.69 13.87,95.4 16.76,95.4 LED2.GREEN_C
N$21
  Bottom 0.152: IC2.19 5.49,104.7 5.49,103.48 6.71,102.26 8.23,102.26 12.34,98.15 LED1.RED_C
N$22  (via drill 0.4)
  Top 0.152: v18.75,90.22 18.75,85.65 v19.2,85.19
  Bottom 0.152: v18.75,90.22 17.22,90.22 14.17,93.27 14.17,93.42 10.36,97.23 7.77,97.23 6.25,98.75 6.25,99.21 IC2.5 | v19.2,85.19 16.92,82.91 16.61,82.91 13.26,79.55 13.26,78.49 LED5.RED_C
N$23
  Bottom 0.152: IC2.20 6.25,104.7 6.25,103.17 6.86,102.56 9.6,102.56 10.06,102.11 11.89,102.11 14.33,99.67 16,99.67 17.53,98.15 LED1.GREEN_C
N$24
  Bottom 0.152: R49.1 18.29,44.81 J3.NORM
N$25
  Bottom 0.152: R48.1 3.05,35.2 5.03,35.2 J2.NORM
N$26
  Bottom 0.152: R45.1 25.15,35.05 24.99,35.2 J4.NORM
N$27  (via drill 0.4)
  Top 0.152: v21.79,99.82 v17.68,99.82
  Bottom 0.152: IC2.24 8.69,104.7 8.99,104.7 10.67,103.02 C8.1 10.67,102.87 11.58,102.87 14.48,99.97 17.53,99.97 v17.68,99.82 | F1.1 C2.+ 22.86,99.82 v21.79,99.82
N$28  (via drill 0.4)
  Top 0.152: v11.89,29.72 11.89,33.53 v11.58,33.83
  Bottom 0.152: v11.89,29.72 11.89,28.19 IC6.6 | v11.58,33.83 11.58,34.44 10.97,35.05 R18.2 C39.1 | C39.1 R26.1 10.97,38.1 11.89,39.01 15.54,39.01 16.46,38.1 R14.1 | C39.1
N$29  (via drill 0.4)
  Top 0.152: v12.95,8.53 v10.21,5.79
  Bottom 0.152: v10.21,5.79 8.99,4.57 4.27,4.57 2.9,5.94 2.9,6.4 J9.A | v12.95,8.53 16.76,8.53 25.76,17.53 25.91,17.53 27.13,18.75 27.13,19.05 J5.C
N$30
  Bottom 0.152: J9.C 7.47,6.55 12.65,6.55 J8.A
N$31
  Bottom 0.152: 2.9,27.74 2.9,28.96 R41.2 | 2.9,27.74 2.9,27.43 C56.1 2.9,27.74 | 2.9,27.74 5.03,27.74 J2.IN
N$32
  Bottom 0.152: J8.C 17.37,6.55 22.55,6.55 J10.A
N$33
  Bottom 0.152: R4.2 14.33,60.5 14.33,55.47 16.31,53.49 16.31,48.31 15.09,47.09 J3.A
N$34
  Bottom 0.152: R5.2 15.85,60.5 15.85,55.17 20.57,50.44 20.57,47.7 19.66,46.79 19.66,39.01 23.62,35.05 23.62,34.9 24.69,33.83 27.13,33.83 28.19,32.77 28.19,31.09 26.98,29.87 25.6,29.87 24.99,29.26 22.4,29.26 16.31,23.16 16.31,22.1 15.24,21.03 14.17,21.03 12.8,19.66 12.8,19.2 J6.A
N$35  (via drill 0.4)
  Top 0.152: v16.92,62.33 16.92,63.7 14.17,66.45 14.17,71.63 14.63,72.08 15.39,72.08 16,71.48 16,68.12 16.46,67.67 17.07,67.67 21.18,71.78 21.18,79.1 23.62,81.53 23.62,99.67 29.11,105.16 29.11,106.22 28.19,107.14 21.79,107.14 JP58.1
  Bottom 0.152: R4.1 14.33,62.33 15.7,62.33 R5.1 15.85,62.33 v16.92,62.33
N$36
  Bottom 0.152: R51.1 15.24,35.05 15.09,35.2 J7.NORM
N$37
  Bottom 0.152: IC6.13 9.3,22.55 9.3,16.61 8.99,16.31 R31.2 8.99,16.15 8.99,14.78 C46.1 8.99,14.63 8.99,13.26 R30.1 8.84,13.11 8.84,11.73 5.64,8.53 3.05,8.53 1.83,7.32 1.83,5.49 3.05,4.27 9.14,4.27 9.3,4.42 17.98,4.42 18.75,3.66 R40.1
N$39
  Bottom 0.152: 8.99,36.58 8.99,35.05 R32.2 8.84,35.05 7.62,33.83 2.13,33.83 0.61,32.31 0.61,31.7 2.13,30.18 | 8.99,36.58 8.99,38.1 R33.1 | 8.99,36.58 C47.1 | 2.13,30.18 3.66,30.18 3.81,30.02 7.92,30.02 9.3,28.65 9.3,28.19 IC6.2 | 2.13,30.18 1.22,29.26 1.22,28.96 R41.1
N$44
  Bottom 0.152: R15.1 12.5,48.77 11.58,49.68 6.71,49.68 JP20.1
N$45  (via drill 0.4)
  Top 0.152: v21.79,52.43 23.01,53.65 23.93,53.65 24.69,54.41 24.69,56.08 25.91,57.3 JP22.1
  Bottom 0.152: v21.79,52.43 21.79,49.68 22.86,48.62 22.86,44.35 27.89,39.32 27.89,34.44 28.65,33.68 28.65,28.96 R39.1
N$49  (via drill 0.4)
  Top 0.152: v2.9,17.68 2.9,19.96 4.27,21.34 5.79,21.34 13.11,28.65 13.72,28.65 14.78,29.72 15.85,29.72 17.22,31.09 17.22,34.75 15.39,36.58 14.48,36.58 13.72,37.34 13.72,38.41 19.66,44.35 19.66,47.85 22.86,51.05 24.69,51.05 25.91,52.27 JP24.1
  Bottom 0.152: v2.9,17.68 1.52,16.31 R38.1
N$50  (via drill 0.4)
  Top 0.152: v28.8,23.62 28.8,24.23 29.41,24.84 29.41,44.04 v28.04,45.41
  Bottom 0.152: v28.8,23.62 28.8,16.31 R13.1 | v28.04,45.41 26.98,46.48 26.98,49.07 27.13,49.23 27.13,53.65 JP26.1
N$52  (via drill 0.4)
  Top 0.152: v13.26,2.13 15.39,4.27 17.68,4.27 24.54,11.12 25.45,11.12 26.06,11.73 26.06,15.39 24.38,17.07 23.93,17.07 22.71,18.29 v22.71,20.73 | v22.71,28.5 22.71,41.76 23.62,42.67 v23.62,46.33
  Bottom 0.152: v13.26,2.13 8.99,2.13 R46.2 | v22.71,28.5 v22.71,20.73 | v23.62,46.33 23.62,49.53 JP54.1
N$53  (via drill 0.4)
  Top 0.152: v28.65,13.56 28.65,22.25 v28.04,22.86 | v28.04,25.76 28.04,35.81 27.89,35.97 v27.89,40.84
  Bottom 0.152: v28.65,13.56 28.65,2.13 R47.2 | v28.04,25.76 v28.04,22.86 | v27.89,40.84 25.91,42.82 JP55.1
N$65
  Bottom 0.152: R46.1 7.16,2.13 5.18,2.13 J9.IN
N$68
  Bottom 0.152: IC2.23 8.08,104.85 8.08,106.38 8.38,106.68 R3.1
N$69
  Bottom 0.152: R47.1 26.98,2.13 24.99,2.13 J10.IN
NORMALIZATION_PROBE  (via drill 0.4)
  Top 0.152: v19.81,50.14 21.18,50.14 JP30.1 | 16.31,16.92 16.31,17.37 17.22,18.29 17.22,21.49 | 17.22,21.49 17.22,22.1 15.54,23.77 14.63,23.77 13.72,24.69 13.72,28.19 14.94,29.41 16,29.41 17.98,31.39 v17.98,33.83 | v1.83,35.66 1.83,32.61 3.05,31.39 3.05,30.33 v4.12,29.26 | v1.83,17.68 2.59,16.92 16.31,16.92 | 16.31,16.92 v16.31,16.61 | v28.65,36.27 28.65,26.21 28.8,26.06 28.8,24.69 25.45,21.34 23.16,21.34 23.01,21.49 17.22,21.49
  Bottom 0.152: R45.2 28.65,35.05 v28.65,36.27 28.65,39.01 24.54,43.13 24.54,51.21 23.47,52.27 JP30.1 23.32,52.43 22.1,53.65 22.1,58.22 20.27,60.05 20.12,60.05 18.9,61.27 D3.3 | v19.81,50.14 18.29,48.62 R49.2 | v16.31,16.61 16.61,16.31 17.37,16.31 R50.1 | v17.98,33.83 19.2,35.05 R51.2 | v1.83,35.66 3.05,36.88 R48.2 | v4.12,29.26 3.5,29.87 2.29,29.87 1.98,29.57 1.98,20.27 1.83,20.12 v1.83,17.68
SW_1
  Top 0.152: SW1.4 1.98,47.09 1.98,47.7 JP47.1 4.12,49.68 6.71,47.09 8.23,47.09 SW1.3
SW_2
  Top 0.152: SW2.4 21.79,47.09 28.04,47.09 SW2.3 28.19,47.09 28.35,47.24 28.35,49.68 JP48.1
TIMBRE_ATT
  Bottom 0.152: C53.1 5.03,62.48 5.03,60.2 R42.2 5.18,60.05 5.33,59.89 5.33,57 6.55,55.78 6.55,54.86 JP45.1
TIMBRE_POT
  Top 0.152: JP42.1 3.96,54.86 3.96,55.78 2.9,56.84 2.9,58.67 3.81,59.59 3.81,73 5.03,74.22 R7.2
  Bottom 0.152: C32.1 5.03,76.66 5.03,74.37 R7.2
V_OCT_IN
  Bottom 0.152: 3.2,14.78 3.2,16.15 R38.2 | 3.2,14.78 5.03,14.78 J1.IN | 3.2,14.78 C60.1

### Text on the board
bPlace: ANTUMBRA / KNIT | WWW.ANTUMBRA.EU | V1.0
tStop: Plaits | cc-by-sa | 2017. v5 | Olivier Gillet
